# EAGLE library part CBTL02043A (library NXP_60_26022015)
CBTL02043A/B is a 2 differential channel, 2-to-1 multiplexer/demultiplexer switch for PCI Express Generation 3 (Gen3), or other high-speed serial interface applications. The CBTL02043A/B can switch two differential signals to one of two locations. Using a unique design technique, NXP has minimized the impedance of the switch such that the attenuation observed through the switch is negligible, and also minimized the channel-to-channel skew as well as channel-to-channel crosstalk, as required by the high-speed serial interface. CBTL02043A/B allows expansion of existing high speed ports for extremely low power. AAL Eindhoven MK
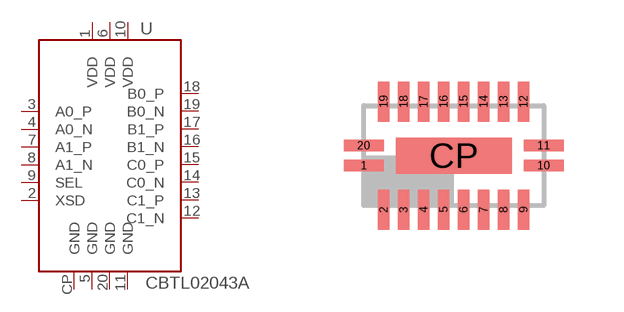
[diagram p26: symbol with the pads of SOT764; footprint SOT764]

Designator prefix U

## CBTL02043ABQ  [SOT764]
1  VDD
2  XSD  in
3  A0_P
4  A0_N
5  GND
6  VDD
7  A1_P
8  A1_N
9  SEL  in
10  VDD
11  GND
12  C1_N
13  C1_P
14  C0_N
15  C0_P
16  B1_N
17  B1_P
18  B0_P
19  B0_N
20  GND
CP  GND

## Footprint SOT764 (pad centres in mm)
SOT764 DHVQFN20: plastic dual in-line compatible thermal enhanced very thin quad flat package; no leads; 20 terminals; body 2.5 x 4.5 x 0.85 mm JEDEC: MO-241 IEC: ---
smd 1 x 0.29: 1 -2.25,-0.25; 10 2.25,-0.25; 11 2.25,0.25; 20 -2.25,0.25
smd 0.29 x 1: 2 -1.75,-1.35; 3 -1.25,-1.35; 4 -0.75,-1.35; 5 -0.25,-1.35; 6 0.25,-1.35; 7 0.75,-1.35; 8 1.25,-1.35; 9 1.75,-1.35; 12 1.75,1.35; 13 1.25,1.35; 14 0.75,1.35; 15 0.25,1.35; 16 -0.25,1.35; 17 -0.75,1.35; 18 -1.25,1.35; 19 -1.75,1.35
smd 2.9 x 0.9: CP 0,0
